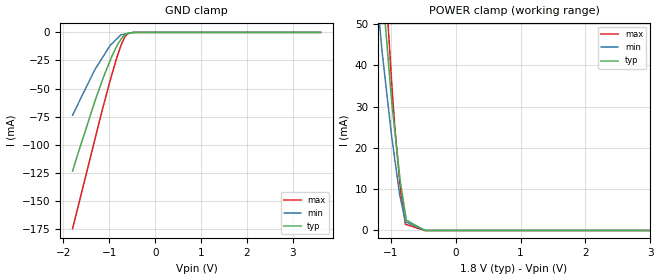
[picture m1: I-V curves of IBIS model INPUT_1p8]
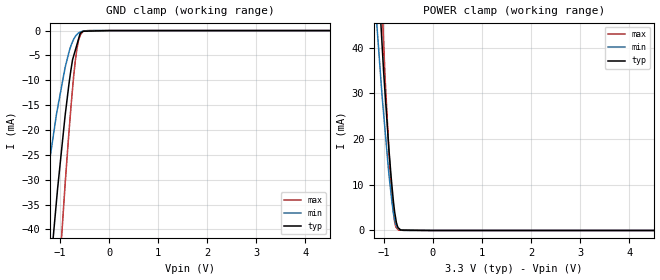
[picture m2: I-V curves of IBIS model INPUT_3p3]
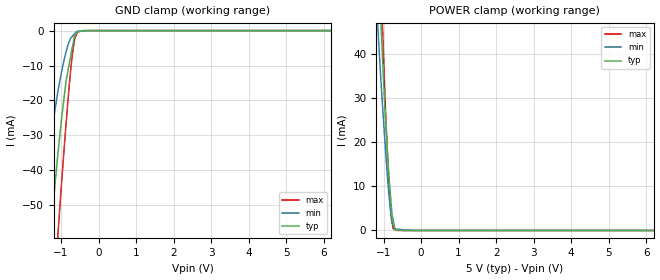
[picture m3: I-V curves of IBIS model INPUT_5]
|Texas Instruments Incorporated
| 16-Bit 250kHz CMOS Analog-to-Digital Converter w/Serial Interface
| 4.096V Internal Reference
| Marketing part#   Digital Voltage Range   Package-type   #pins
| ADS8519IBDB   1.65V - 5.25V   SSOP   28
| ADS8519IBDBG4   1.65V - 5.25V   SSOP   28
| ADS8519IBDBR   1.65V - 5.25V   SSOP   28
| ADS8519IBDBRG4   1.65V - 5.25V   SSOP   28
| ADS8519IDB   1.65V - 5.25V   SSOP   28
| ADS8519IDBG4   1.65V - 5.25V   SSOP   28
| ADS8519IDBR   1.65V - 5.25V   SSOP   28
| ADS8519IDBRG4   1.65V - 5.25V   SSOP   28
[IBIS Ver]   3.2
[File name]   ads8519.ibs
|SIMDE Ver   V2.2 - 201009 - RHL4 - Build 424
[File Rev]   1.1
[Date]   02/10/2011
[Source]
| Texas Instruments Incorporated.
| Analog-eLab Design Center, HPA
| 12500 TI Blvd
| Dallas, TX -75243
| e-mail: elab_ibis@list.ti.com
| -Model generated from simulations in TISPICE
[Notes]   Revision History:
| Rev 1.0: 12/13/2010
| - Initial version of the model
| - Model generated from simulations in TISPICE
| - Model matched to SPICE simulation
| - C_comp although listed in numerical order of value are
|   obtained from varying PVT conditions. For PVT conditions for
|   each specific value refer the buffer description under
|   respective [Model]. IBIS model user is responsible for using
|   appropriate C_comp to simulate for Signal Integrity.
| - Model names with a trailing 1p8 contains the model for
|   1.8V [1.71V and 1.89V].Model names with a trailing 3p3 contains
|   the model for 3.3V [3.0V and 3.6V]. Model names with trailing 5
|   contains the model for 5.0V [4.75V and 5.25V] operation.
| Rev 1.1:01/07/2011
| - Updated with C_Comp measurment frequency and L value for LC
|   tank.
| Rev 1.2:02/102011
| - Updated file, removing references to ADS8515 and correcting title
[Disclaimer]
| This model is designed as an aid for customers of Texas Instruments.
| TI and its licensors and suppliers make no warranties, either expressed
| or implied, with respect to this  model, including the warranties of
| merchantability or fitness for a particular purpose. The model is
| provided solely on an "as is" basis. The entire risk as to its quality
| and performance is with the customer.
[Copyright]
 (C) Copyright 2010 Texas Instruments Incorporated.All rights reserved.
|   ADS8519
[Component]   ADS8519
[Manufacturer]   TI
[Package]   |28 SSOP -  DB package
|   typ   min   max
R_pkg   0.11526   0.04806   0.14207
L_pkg   2.88484nH   1.68796nH   4.11905nH
C_pkg   0.48438pF   0.37109pF   0.64184pF
[Pin]  signal_name   model_name   R_pin   L_pin   C_pin
1   R1IN   TERM   0.14207   4.11905nH  0.61829pF
2   AGND1   GND   0.07467   3.13764nH  0.64747pF
3   R2IN   TERM   0.13555   3.23217nH  0.49118pF
4   R3IN   TERM   0.12314   2.44151nH  0.39417pF
5   NC   NC   0.00537   1.05191nH  0.33021pF
6   CAP   TERM   0.04806   1.68796nH  0.40937pF
7   REF   TERM   0.08687   1.90164nH  0.37382pF
8   NC   NC   0.00526   1.01905nH  0.31614pF
9   AGND2   GND   0.04502   1.58088nH  0.40485pF
10   NC   NC   0.00537   1.05288nH  0.33025pF
11   NC   NC   0.00542   1.07612nH  0.31412pF
12   SB/_BTC   INPUT   0.13353   3.20369nH  0.48596pF
13   EXT/_INT   INPUT   0.13633   3.59505nH  0.59548pF
14   DGND   GND   0.14068   4.10650nH  0.61387pF
15   SYNC   DATA_SYNC   0.14062   4.10570nH  0.61392pF
16   DATACLK   DATACLK   0.13641   3.59615nH  0.59569pF
17   DATA   DATA_SYNC   0.13381   3.20759nH  0.48650pF
18   NC   NC   0.00542   1.07612nH  0.31412pF
19   TAG   INPUT   0.09650   2.06488nH  0.39000pF
20   NC   NC   0.00532   1.03496nH  0.32320pF
21   R/_C   INPUT   0.08919   1.93341nH  0.37109pF
22   NC   NC   0.00526   1.01882nH  0.31622pF
23   NC   NC   0.00531   1.03451nH  0.32329pF
24   _CS   INPUT   0.10716   2.20361nH  0.39674pF
25   _BUSY   BUSY   0.12396   2.45281nH  0.39595pF
26   PWRD   INPUT   0.13536   3.22957nH  0.49008pF
27   VANA   TERM   0.07553   3.18269nH  0.64184pF
28   VDIG   POWER   0.14556   4.16765nH  0.61952pF
|   Model Selectors
[Model Selector] INPUT
INPUT_1p8   1.8V digital input
INPUT_3p3   3.3V digital input
INPUT_5   5.0V digital input
[Model Selector] DATA_SYNC
data_sync_1p8   1.8V digital output
data_sync_3p3   3.3V digital output
data_sync_5   5.0V digital output
[Model Selector] BUSY
busy_1p8   1.8V digital output
busy_3p3   3.3V digital output
busy_5   5.0V digital output
[Model Selector] DATACLK
DATACLK_1p8   1.8V digital I/O
DATACLK_3p3   3.3V digital I/O
DATACLK_5   5.0V digital I/O
[Model Selector] TERM
TERM_1p8   1.8V nominal termination
TERM_3p3   3.3V nominal termination
TERM_5   5.0V nominal termination
[Model]  TERM_1p8
Model_type Terminator
C_comp   1.0e-20F  1.0e-20F  1.0e-20F
|   typ   min   max
[Voltage Range]   1.8V   1.71V   1.89V
[POWER Clamp Reference]   1.8V   1.71V   1.89V
[GND Clamp Reference]   0V   0V   0V
|Ambient Temperature   25   85   -40
|Junction Temperature
[Temperature Range]   32   92   -40
[Model]  TERM_3p3
Model_type Terminator
C_comp   1.0e-20F  1.0e-20F  1.0e-20F
|   typ   min   max
[Voltage Range]   3.3V   3.0V   3.6V
[POWER Clamp Reference]   3.3V   3.0V   3.6V
[GND Clamp Reference]   0V   0V   0V
|Ambient Temperature   25   85   -40
|Junction Temperature
[Temperature Range]   32   92   -40
[Model]  TERM_5
Model_type Terminator
C_comp   1.0e-20F  1.0e-20F  1.0e-20F
|   typ   min   max
[Voltage Range]   5.0V   4.75V   5.25V
[POWER Clamp Reference]   5.0V   4.75V   5.25V
[GND Clamp Reference]   0V   0V   0V
|Ambient Temperature   25   85   -40
|Junction Temperature
[Temperature Range]   32   92   -40
| Models and submodels in the file (15): INPUT_1p8 (Input), INPUT_3p3 (Input), INPUT_5 (Input), DATACLK_1p8 (I/O), DATACLK_3p3 (I/O), DATACLK_5 (I/O), data_sync_1p8 (Output), data_sync_3p3 (Output), data_sync_5 (Output), busy_1p8 (Output), busy_3p3 (Output), busy_5 (Output), TERM_1p8 (Terminator), TERM_3p3 (Terminator), TERM_5 (Terminator)
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|   input_1p8 Model
[Model]   INPUT_1p8
Model_type   Input
Vinl = 0.6
Vinh = 0.9
|   typ   min   max
|   (nom PVT)   (Fast PVT)   (slow PVT)
| C_comp by Frequency Method (F=29Mhz)
| C_comp   7.637e-12   8.292e-12   6.875e-12
| C_comp by LC tank Method (L=1nH)
| Resonant frequency (Hz)  1.93e9   1.99e9   1.88e9
C_comp   6.807e-12   6.403e-12   7.174e-12
| Where nom  PVT is Nominal Process,  1.8V,  32C
|   Fast PVT is Strong Process,   1.89V,  -40C
|   Slow PVT is Weak Process,   1.71V,  92C
[Model Spec]
Vinl   0.6   0.6   0.6
Vinh   0.9   0.855   0.945
[Voltage Range]   1.8   1.71   1.89
|Ambient Temperature   25   85   -40
|Junction Temperature
[Temperature Range]   32   92   -40
[Power Clamp Reference]   1.8   1.71   1.89
[GND Clamp Reference]   0   0   0
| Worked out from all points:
|   GND clamp passes 1 mA (typ) near -0.61 V on its own axis
[GND Clamp]
|   Voltage   I(typ)   I(min)   I(max)
-1.8V     -123.6mA   -73.74mA   -174.9mA
-1.318V   -61.94mA   -33.52mA   -96.05mA
-1.114V   -38.5mA    -20.2mA    -63.27mA
-981.5mV  -25.08mA   -11.55mA   -42.97mA
-945mV    -21.38mA   -10.08mA   -37.64mA
-811.8mV  -10.19mA   -4.81mA    -19.66mA
-733.3mV  -5.47mA    -2.091mA   -10.22mA
-702mV    -3.614mA   -1.846mA   -7.527mA
-657.7mV  -2.301mA   -1.499mA   -3.727mA
-584mV    -659.1uA   -921.8uA   -803uA
-412.1mV  -6.485uA   -6.835uA   -4.049uA
3.6V      0A         0A         0A
[POWER Clamp]
|   Voltage   I(typ)   I(min)   I(max)
-1.8V     223.4mA    177mA      278.6mA
-1.2V     75.98mA    55.01mA    95.19mA
-1.132V   60.64mA    43.28mA    75.57mA
-1.096V   52.57mA    38.28mA    65.25mA
-1.045V   42.85mA    31.16mA    51.25mA
-981mV    30.72mA    22.38mA    34.97mA
-937.4mV  24.32mA    17.36mA    25.25mA
-846.7mV  11.31mA    7.583mA    9.265mA
-773mV    4.008mA    2.095mA    1.491mA
-757.8mV  2.501mA    1.984mA    1.416mA
-471.6mV  95.85nA    9.602uA    4.882uA
3.6V      0A         0A         0A
|   input_3p3 Model
[Model]   INPUT_3p3
Model_type   Input
Vinl = 0.6
Vinh = 1.65
|   typ   min   max
|   (nom PVT)   (Fast PVT)   (slow PVT)
| C_comp by Frequency Method(F=29Mhz)
| C_comp   6.589e-12   5.841e-12   7.284e-12
| C_comp by LC tank Method (L=1nH)
| Resonant frequency (Hz)  2.07e9   2.16e9   2.0e9
C_comp   5.918e-12   5.435e-12   6.339e-12
| Where nom  PVT is Nominal Process,  3.3V,  32C
|   Fast PVT is Strong Process,   3.6V,  -40C
|   Slow PVT is Weak Process,   3.0V,  92C
[Model Spec]
Vinl   0.6   0.6   0.6
Vinh   1.65   1.5   1.85
[Voltage Range]   3.3   3   3.6
|Ambient Temperature   25   85   -40
|Junction Temperature
[Temperature Range]   32   92   -40
[Power Clamp Reference]   3.3   3   3.6
[GND Clamp Reference]   0   0   0
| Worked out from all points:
|   GND clamp passes 1 mA (typ) near -0.60 V on its own axis
|   POWER clamp passes 1 mA (typ) near -0.72 V on its own axis
[GND Clamp]
|   Voltage   I(typ)   I(min)   I(max)
-3.3V     -333mA     -232.2mA   -422.8mA
-1.435V   -76.21mA   -42.84mA   -114.7mA
-1.382V   -69.81mA   -38.69mA   -106mA
-1.231V   -51.56mA   -27.35mA   -81.58mA
-1.102V   -37.36mA   -18.69mA   -61.11mA
-1.053V   -31.99mA   -15.7mA    -53.88mA
-897.6mV  -17.1mA    -7.418mA   -30.93mA
-782.1mV  -8.111mA   -3.138mA   -15.8mA
-684mV    -3.747mA   -1.087mA   -5.602mA
-591mV    -576uA     -301.1uA   -1.019mA
-378mV    -95.05uA   -2.622uA   -1.144uA
6.6V      0A         0A         0A
[POWER Clamp]
|   Voltage   I(typ)   I(min)   I(max)
-3.3V     609.2mA    511mA      750.6mA
-1.155V   65.36mA    46.91mA    83.01mA
-1.102V   53.84mA    39.19mA    67.43mA
-1.069V   47mA       34.36mA    57.76mA
-1.035V   40.53mA    29.35mA    48.96mA
-1.003V   34.52mA    25.43mA    40.78mA
-975.6mV  30.18mA    22.02mA    33.68mA
-896.4mV  17.76mA    12.27mA    17.36mA
-838.8mV  10.25mA    6.592mA    8.136mA
-774mV    3.682mA    2.138mA    1.546mA
-702mV    537.3uA    340uA      63.57uA
6.6V      0A         0A         0A
|   input_5 Model
[Model]   INPUT_5
Model_type   Input
Vinl = 0.6
Vinh = 2.5
|   typ   min   max
|   (nom PVT)   (Fast PVT)   (slow PVT)
| C_comp by Frequency Method(F=29Mhz)
| C_comp   5.827e-12   5.209e-12   6.392e-12
| C_comp by LC tank Method (L=1nH)
| Resonant frequency (Hz)  2.2e9   2.28e9   2.13e9
C_comp   5.239e-12   4.878e-12   5.589e-12
| Where nom  PVT is Nominal Process,  5V,  32C
|   Fast PVT is Strong Process,   5.25V,  -40C
|   Slow PVT is Weak Process,   4.75V,  92C
[Model Spec]
Vinl   0.6   0.6   0.6
Vinh   2.5   2.375   2.625
[Voltage Range]   5   4.75   5.25
|Ambient Temperature   25   85   -40
|Junction Temperature
[Temperature Range]   32   92   -40
[Power Clamp Reference]   5   4.75   5.25
[GND Clamp Reference]   0   0   0
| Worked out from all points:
|   GND clamp passes 1 mA (typ) near -0.61 V on its own axis
|   POWER clamp passes 1 mA (typ) near -0.71 V on its own axis
[GND Clamp]
|   Voltage   I(typ)   I(min)   I(max)
-5V       -574.5mA   -430.2mA   -701.3mA
-1.72V    -112.9mA   -67.43mA   -161.9mA
-1.558V   -91.86mA   -52.81mA   -135.2mA
-1.306V   -60.44mA   -32.61mA   -93.6mA
-1.145V   -42.11mA   -21.56mA   -67.79mA
-1.08V    -34.84mA   -17.23mA   -57.9mA
-865mV    -14.34mA   -6.09mA    -26.59mA
-729.8mV  -6.596mA   -2.001mA   -9.841mA
-640.5mV  -1.489mA   -939.9uA   -2.745mA
-570mV    -359.4uA   -216.3uA   -657.9uA
-388.5mV  -5.808uA   -113uA     -1.69uA
10V       0A         0A         0A
[POWER Clamp]
|   Voltage   I(typ)   I(min)   I(max)
-5V       1.051A     894.9mA    1.289A
-1.216V   79.7mA     57.28mA    100.4mA
-1.14V    62.03mA    44.52mA    78.12mA
-1.054V   44.45mA    32mA       53.93mA
-1.018V   37.73mA    27.33mA    44.25mA
-950.3mV  25.75mA    18.5mA     27.96mA
-897.8mV  18.19mA    12.41mA    17.6mA
-829.5mV  9.475mA    5.828mA    6.879mA
-787.5mV  5.021mA    3.019mA    2.439mA
-740.2mV  2.252mA    1.189mA    385uA
-640.5mV  53.47uA    307.2uA    3.245uA
10V       0A         0A         0A
